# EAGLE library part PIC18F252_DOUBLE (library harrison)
PIC18F252 Microcontroller with bothZIF 28-6 and DIP 28-3 sockets
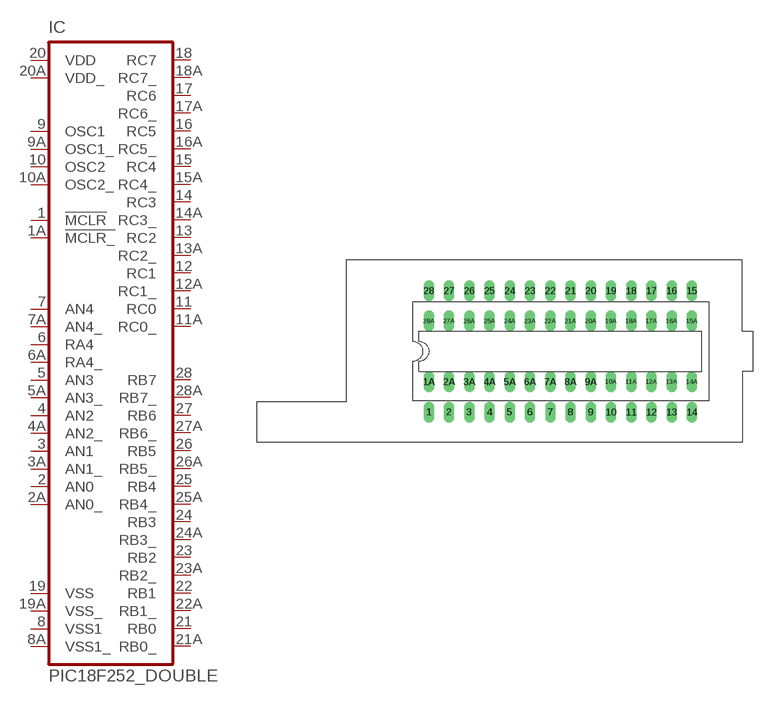
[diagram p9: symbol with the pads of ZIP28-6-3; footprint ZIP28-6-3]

Designator prefix IC

## PIC18F252_DOUBLE  [ZIP28-6-3]
1  !MCLR  in
1A  !MCLR_  in
2  AN0
2A  AN0_
3  AN1
3A  AN1_
4  AN2
4A  AN2_
5  AN3
5A  AN3_
6  RA4
6A  RA4_
7  AN4
7A  AN4_
8  VSS1  pwr
8A  VSS1_  pwr
9  OSC1
9A  OSC1_
10  OSC2
10A  OSC2_
11  RC0
11A  RC0_
12  RC1
12A  RC1_
13  RC2
13A  RC2_
14  RC3
14A  RC3_
15  RC4
15A  RC4_
16  RC5
16A  RC5_
17  RC6
17A  RC6_
18  RC7
18A  RC7_
19  VSS  pwr
19A  VSS_  pwr
20  VDD  pwr
20A  VDD_  pwr
21  RB0
21A  RB0_
22  RB1
22A  RB1_
23  RB2
23A  RB2_
24  RB3
24A  RB3_
25  RB4
25A  RB4_
26  RB5
26A  RB5_
27  RB6
27A  RB6_
28  RB7
28A  RB7_

## Footprint ZIP28-6-3 (pad centres in mm)
drill 0.813 long: 1 -15.24,-7.62; 1A -15.24,-3.81; 2 -12.7,-7.62; 2A -12.7,-3.81; 3 -10.16,-7.62; 3A -10.16,-3.81; 4 -7.62,-7.62; 4A -7.62,-3.81; 5 -5.08,-7.62; 5A -5.08,-3.81; 6 -2.54,-7.62; 6A -2.54,-3.81; 7 0,-7.62; 7A 0,-3.81; 8 2.54,-7.62; 8A 2.54,-3.81; 9 5.08,-7.62; 9A 5.08,-3.81; 10 7.62,-7.62; 10A 7.62,-3.81; 11 10.16,-7.62; 11A 10.16,-3.81; 12 12.7,-7.62; 12A 12.7,-3.81; 13 15.24,-7.62; 13A 15.24,-3.81; 14 17.78,-7.62; 14A 17.78,-3.81; 15 17.78,7.62; 15A 17.78,3.81; 16 15.24,7.62; 16A 15.24,3.81; 17 12.7,7.62; 17A 12.7,3.81; 18 10.16,7.62; 18A 10.16,3.81; 19 7.62,7.62; 19A 7.62,3.81; 20 5.08,7.62; 20A 5.08,3.81; 21 2.54,7.62; 21A 2.54,3.81; 22 0,7.62; 22A 0,3.81; 23 -2.54,7.62; 23A -2.54,3.81; 24 -5.08,7.62; 24A -5.08,3.81; 25 -7.62,7.62; 25A -7.62,3.81; 26 -10.16,7.62; 26A -10.16,3.81; 27 -12.7,7.62; 27A -12.7,3.81; 28 -15.24,7.62; 28A -15.24,3.81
